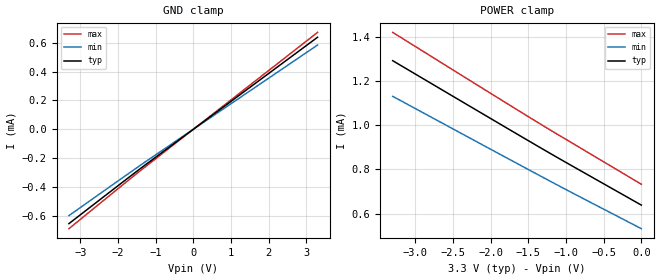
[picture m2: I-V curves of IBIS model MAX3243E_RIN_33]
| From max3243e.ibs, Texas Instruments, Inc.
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[Model]   MAX3243E_RIN_33
Model_type  Input
Vinl=0.8
Vinh=2.0
| variable   typ   min   max
C_comp   1.00pF   1.00pF   1.00pF
[Temperature Range]   40   100   -40
| Ambient temperature   25   85   -40
[Voltage range]   3.3   3   3.6
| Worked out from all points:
|   POWER clamp passes 1 mA (typ) near -1.84 V on its own axis
[GND Clamp]
| MAX3243E_RIN_33
|   Voltage   I(typ)   I(min)   I(max)
-3.3V     -653.8uA   -598.2uA   -688.7uA
-2.025V   -396.5uA   -363uA     -417.4uA
-1.435V   -278.3uA   -254.9uA   -292.9uA
3.3V      638.3uA    584.5uA    671.9uA
[POWER Clamp]
| MAX3243E_RIN_33
|   Voltage   I(typ)   I(min)   I(max)
-3.3V     1.294mA    1.132mA    1.422mA
-1.395V   909.8uA    780.6uA    1.018mA
-915mV    815.4uA    693.6uA    919.3uA
-48.03fV  638.3uA    531.3uA    733uA
